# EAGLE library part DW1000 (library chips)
Description: The DecaWave DW1000 chip, used for UWB two-way ranging.
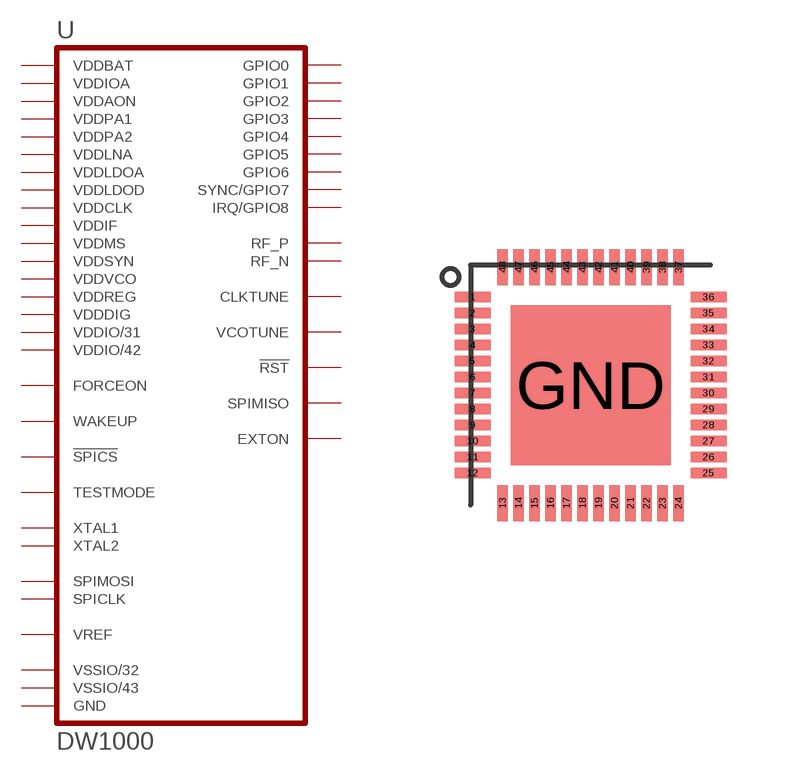
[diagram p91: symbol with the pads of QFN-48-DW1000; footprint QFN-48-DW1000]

Designator prefix U

## DW1000 (DATASHEET: https://www.decawave.com/sites/default/files/resources/dw1000-datasheet-v2.13.pdf; DESCRIPTION: IC RF TXRX 802.15.4 48-QFN; DIGIKEY: 1479-1001-1-ND; MANUFACTURER: Decawave Limited; MPN: DW1000-I-TR13)  [QFN-48-DW1000]
3  XTAL1  in
4  XTAL2  in
5  VREF
6  VDDMS  pwr
7  VDDIF  pwr
8  CLKTUNE
9  VDDCLK  pwr
10  VDDSYN  pwr
11  VDDVCO  pwr
12  VCOTUNE
15  VDDLNA  pwr
16  RF_P
17  RF_N
18  VDDPA1  pwr
19  VDDPA2  pwr
20  VDDREG  pwr
21  EXTON  out
22  FORCEON  in
23  WAKEUP  in
24  !SPICS  in
25  VDDAON  pwr
26  VDDLDOD  pwr
27  !RST
28  VDDIOA  pwr
29  SYNC/GPIO7
30  GPIO6
31  VDDIO/31  pwr
32  VSSIO/32
33  GPIO5
34  GPIO4
35  GPIO3
36  GPIO2
37  GPIO1
38  GPIO0
39  SPIMOSI  in
40  SPIMISO  out
41  SPICLK  in
42  VDDIO/42  pwr
43  VSSIO/43
44  VDDDIG  pwr
45  IRQ/GPIO8
46  TESTMODE  in
47  VDDBAT  pwr
48  VDDLDOA  pwr
GND  GND  pwr

## Footprint QFN-48-DW1000 (pad centres in mm)
Description: Footprint for the DW1000, designed based on the previous version of TriPoint available on Github.
smd 0.9 x 0.26: 1 -2.95,2.2; 2 -2.95,1.8; 3 -2.95,1.4; 4 -2.95,1; 5 -2.95,0.6; 6 -2.95,0.2; 7 -2.95,-0.2; 8 -2.95,-0.6; 9 -2.95,-1; 10 -2.95,-1.4; 11 -2.95,-1.8; 12 -2.95,-2.2; 25 2.95,-2.2; 26 2.95,-1.8; 27 2.95,-1.4; 28 2.95,-1; 29 2.95,-0.6; 30 2.95,-0.2; 31 2.95,0.2; 32 2.95,0.6; 33 2.95,1; 34 2.95,1.4; 35 2.95,1.8; 36 2.95,2.2
smd 0.26 x 0.9: 13 -2.2,-2.95; 14 -1.8,-2.95; 15 -1.4,-2.95; 16 -1,-2.95; 17 -0.6,-2.95; 18 -0.2,-2.95; 19 0.2,-2.95; 20 0.6,-2.95; 21 1,-2.95; 22 1.4,-2.95; 23 1.8,-2.95; 24 2.2,-2.95; 37 2.2,2.95; 38 1.8,2.95; 39 1.4,2.95; 40 1,2.95; 41 0.6,2.95; 42 0.2,2.95; 43 -0.2,2.95; 44 -0.6,2.95; 45 -1,2.95; 46 -1.4,2.95; 47 -1.8,2.95; 48 -2.2,2.95
smd 4 x 4: GND 0,0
